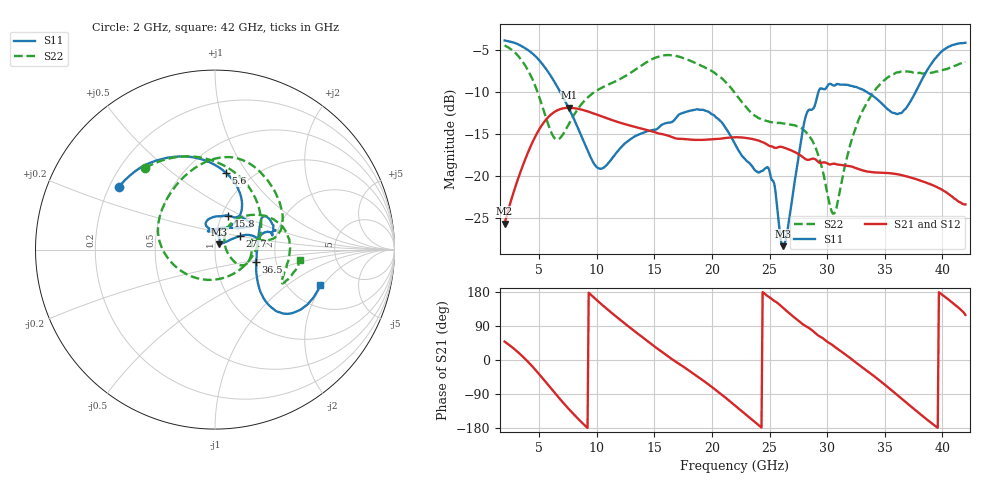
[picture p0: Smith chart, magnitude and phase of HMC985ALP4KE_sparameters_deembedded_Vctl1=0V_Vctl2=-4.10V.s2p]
!s2p File: Measurements: S11, S21, S12, S22
# GHz S dB R 50.0
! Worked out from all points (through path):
!   401 points, 2 GHz to 42 GHz, reference 50 ohm
!   highest |S21| = -11.90 dB at 7.6 GHz (marker M1); lowest = -25.7 dB at 2 GHz (marker M2)
!   lowest |S11| = -28.4 dB at 26.2 GHz (marker M3), VSWR 1.08, Z = 52.3 + j3.17 ohm
!   |S11| at or under -10 dB: 6.821 GHz to 29.25 GHz (22.43 GHz wide, 124 % of centre); 33.42 GHz to 37.69 GHz (4.27 GHz wide, 12 % of centre)
!   |S22| runs from -24.5 to -4.5 dB; largest |S21 - S12| = 0.00023
!   S11 on the Smith chart (normalised r, x): 2 GHz: 0.24, +0.28; 5.6 GHz: 0.76, +0.80; 15.8 GHz: 1.07, +0.42; 27.7 GHz: 1.30, +0.20; 36.5 GHz: 1.57, -0.23; 42 GHz: 2.95, -1.89
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2  -3.88 147.0  -25.67 48.6  -25.67 48.6  -4.47 130.5
3.6  -4.66 120.3  -18.70 8.3  -18.70 8.3  -6.48 84.9
4.7  -5.80 99.5  -15.22 -26.9  -15.22 -26.9  -9.44 43.4
5.6  -7.28 81.9  -13.29 -59.2  -13.30 -59.2  -13.10 -3.8
6.5  -9.22 66.5  -12.25 -92.1  -12.25 -92.1  -15.66 -69.3
7.6  -12.03 54.8  -11.90 -130.2  -11.90 -130.3  -13.76 -136.2
8.7  -15.38 55.0  -12.12 -164.9  -12.12 -164.9  -11.42 -170.5
10.4  -19.14 89.6  -12.90 147.3  -12.90 147.3  -9.53 162.2
15.4  -14.22 75.7  -14.97 27.2  -14.97 27.2  -5.79 86.7
15.8  -13.82 68.7  -15.07 18.3  -15.07 18.2  -5.66 81.6
19.4  -12.23 33.3  -15.71 -57.8  -15.71 -57.8  -7.10 34.6
22  -16.19 51.2  -15.40 -120.1  -15.41 -120.1  -10.15 10.0
24.9  -19.04 104.7  -16.37 167.2  -16.38 167.2  -13.52 13.2
26.2  -28.37 52.5  -16.61 136.8  -16.62 136.8  -13.77 -3.0
27.7  -16.12 28.7  -17.57 98.7  -17.57 98.7  -14.28 -24.0
28.7  -12.11 12.6  -17.96 78.2  -17.96 78.1  -15.77 -32.0
30.6  -9.26 19.5  -18.55 36.2  -18.55 36.2  -24.48 19.3
32.8  -9.59 33.9  -19.23 -13.7  -19.23 -13.7  -13.09 52.7
35.4  -12.22 11.7  -19.68 -75.0  -19.68 -75.0  -8.16 20.7
36.5  -12.47 -16.7  -19.92 -102.9  -19.93 -102.9  -7.58 6.7
39.5  -5.86 -43.7  -21.31 -176.6  -21.31 -176.6  -7.58 -26.2
42  -4.15 -18.5  -23.39 119.0  -23.40 118.9  -6.42 -6.9
